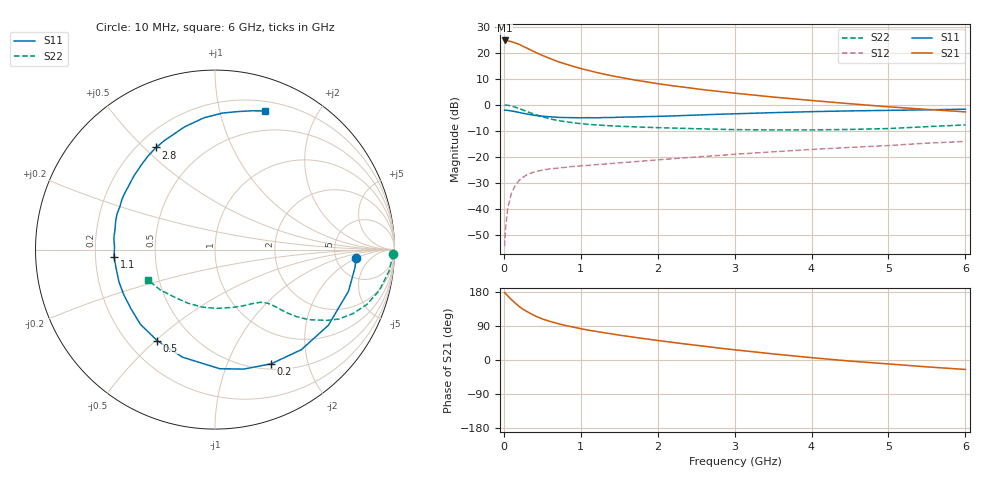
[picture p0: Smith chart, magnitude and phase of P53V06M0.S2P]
! SIEMENS Small Signal Semiconductors
! BFP183
! Si NPN RF Bipolar Junction Transistor in SOT143
! VCE = 3 V  IC = 6 mA
! Common Emitter S-Parameters:  March  1996
# GHz  S  MA  R  50
!  f  S11  S21  S12  S22
! GHz  MAG  ANG  MAG  ANG  MAG  ANG  MAG  ANG
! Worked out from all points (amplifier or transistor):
!   36 points, 10 MHz to 6 GHz, reference 50 ohm
!   highest |S21| = 24.8 dB at 10 MHz (marker M1)
!   |S21| within 3 dB of that: start of sweep to 303.1 MHz
!   unconditionally stable (mu >= 1): 1.45 GHz to 5.605 GHz
!   at 250 MHz: K = 0.23, MSG = 25.2 dB, |S12| = -27.9 dB
!   at 1.4 GHz: K = 0.99, MSG = 16.9 dB, |S12| = -22.6 dB
!   at 6 GHz: K = 0.94, MSG = 5.7 dB, |S12| = -14.1 dB
!   lowest NFmin = 1.20 dB at 450 MHz
!   S11 on the Smith chart (normalised r, x): 10 MHz: 7.85, -1.97; 200 MHz: 0.57, -1.45; 500 MHz: 0.32, -0.51; 1.1 GHz: 0.28, -0.03; 2.8 GHz: 0.27, +0.54; 6 GHz: 0.29, +1.39
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0.01  0.7862 -3.5  17.28 178.0  0.0019 90.2  0.9909 -1.4
0.02  0.7867 -7.0  17.12 176.1  0.0039 86.5  0.988 -2.9
0.05  0.7793 -17.2  17.04 169.3  0.0103 83.1  0.9767 -7.1
0.1  0.7595 -33.7  16.34 159.2  0.0199 72.6  0.9434 -14.0
0.15  0.7365 -49.2  15.43 149.8  0.0283 65.8  0.8986 -20.0
0.2  0.7091 -63.8  14.5 141.2  0.0353 60.2  0.8457 -25.0
0.25  0.6849 -76.4  13.32 133.8  0.0403 54.7  0.791 -29.3
0.3  0.6644 -87.7  12.29 127.9  0.045 50.6  0.7379 -32.3
0.4  0.6261 -106.8  10.43 116.9  0.0512 44.2  0.6536 -36.7
0.5  0.6009 -122.4  8.898 108.4  0.0552 39.8  0.5866 -39.5
0.6  0.5883 -134.8  7.788 101.8  0.0585 37.3  0.5358 -41.2
0.7  0.5727 -144.8  6.793 96.3  0.0604 35.4  0.499 -42.3
0.8  0.567 -154.0  6.099 91.1  0.0625 34.2  0.4727 -43.1
1.1  0.5642 -175.7  4.579 78.7  0.0684 33.6  0.4199 -45.5
1.5  0.5755 164.2  3.396 65.6  0.0762 33.8  0.3858 -49.5
1.8  0.5894 151.6  2.842 57.0  0.0823 34.3  0.3706 -53.7
2.2  0.6106 137.7  2.314 46.3  0.0916 34.6  0.3559 -60.2
2.8  0.6569 120.0  1.802 31.4  0.106 34.0  0.3374 -72.2
3.5  0.7046 103.9  1.409 16.1  0.1242 32.1  0.3278 -88.9
4.5  0.762 86.8  1.046 -2.9  0.151 27.1  0.3352 -117.6
5.5  0.8002 75.1  0.814 -18.1  0.1827 21.5  0.3788 -143.6
6  0.822 70.0  0.73 -25.0  0.1969 17.5  0.4096 -155.6
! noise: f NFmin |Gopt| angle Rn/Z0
0.45  1.2  0.21  41  0.24
0.9  1.25  0.24  101  0.21
1.8  2  0.32  175  0.14
